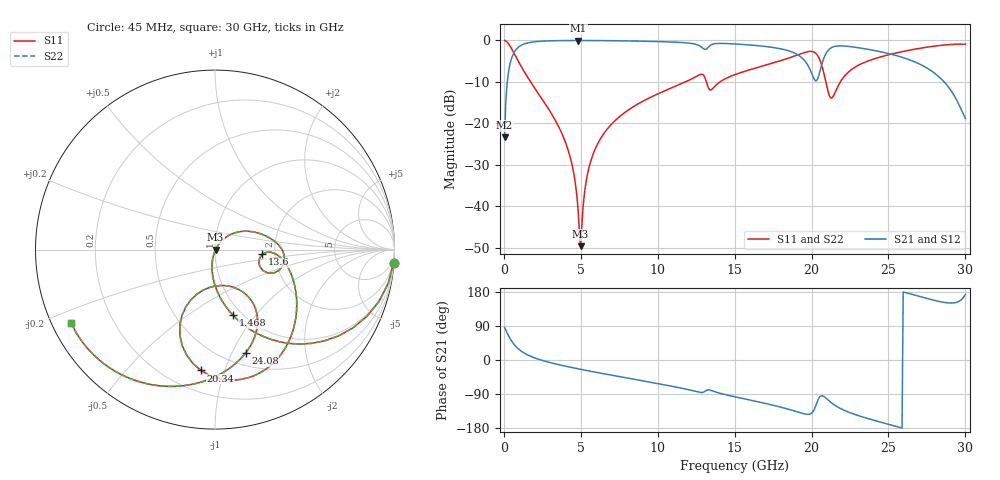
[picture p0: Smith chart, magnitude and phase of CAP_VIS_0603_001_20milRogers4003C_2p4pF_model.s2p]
! S-parameter model data by Modelithics Inc.  support@modelithics.com  813-866-6335  Tampa FL USA
! S-Parameter data specifications:
! Substrate: 20-mil Rogers 4003C, substrate thickness, H=0.508mm, Dielectric constant, Er=3.75
! PCB Mounting Pad Footprint: Pad width, PadW=0.90mm , Pad length, PadL=1.00mm , Pad gap, PadG (edge-to-edge)=1.00mm , Reference planes=3.0mm apart
! Created Wed Nov 18 13:20:45 2015
# hz S ma R 50
! 2 Port Network Data from SP1.SP block
! freq  magS11  angS11  magS21  angS21  magS12  angS12  magS22  angS22
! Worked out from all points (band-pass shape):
!   401 points, 45 MHz to 30 GHz, reference 50 ohm
!   highest |S21| = -0.03 dB at 4.838 GHz (marker M1); lowest = -23.3 dB at 45 MHz (marker M2)
!   |S21| within 3 dB of the highest: 643.6 MHz to 18.88 GHz (18.24 GHz wide, 187 % of centre); 20.96 GHz to 24.84 GHz (3.883 GHz wide, 17 % of centre)
!   lowest |S11| = -49.6 dB at 4.988 GHz (marker M3), VSWR 1.01, Z = 50.3 - j0.0744 ohm
!   |S11| at or under -10 dB: 1.735 GHz to 11.8 GHz (10.07 GHz wide, 149 % of centre); 13.16 GHz to 14.05 GHz (882 MHz wide, 6.48 % of centre); 20.93 GHz to 21.87 GHz (945 MHz wide, 4.42 % of centre)
!   |S22| runs from -49.6 to 0.0 dB; largest |S21 - S12| = 0
!   S11 on the Smith chart (normalised r, x): 45 MHz: 1, -28; 1.468 GHz: 0.91, -0.77; 13.6 GHz: 1.72, -0.10; 20.34 GHz: 0.33, -0.83; 24.08 GHz: 0.63, -1.13; 30 GHz: 0.06, -0.24
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4.5e7  0.9977 -4.1  0.0684 85.9  0.0684 85.9  0.9977 -4.1
4.94325e8  0.7957 -39.7  0.605 50.3  0.605 50.3  0.7957 -39.7
1.467862e9  0.3786 -74.7  0.9238 15.0  0.9238 15.0  0.3786 -74.7
4.014038e9  0.05835 -103.6  0.9951 -16.4  0.9951 -16.4  0.05835 -103.6
4.53825e9  0.02519 -103.8  0.9962 -20.9  0.9962 -20.9  0.02519 -103.8
4.8378e9  0.008286 -90.6  0.9963 -23.3  0.9963 -23.3  0.008286 -90.6
4.987575e9  0.003329 -12.8  0.9963 -24.6  0.9963 -24.6  0.003329 -12.8
5.062462e9  0.005781 30.2  0.9963 -25.2  0.9963 -25.2  0.005781 30.2
5.511788e9  0.02847 54.3  0.9957 -28.7  0.9957 -28.7  0.02847 54.3
6.260662e9  0.06467 52.2  0.9936 -34.5  0.9936 -34.5  0.06467 52.2
1.007992e10  0.2301 25.6  0.9663 -62.9  0.9663 -62.9  0.2301 25.6
1.277588e10  0.3894 -6.7  0.8472 -85.5  0.8472 -85.5  0.3894 -6.7
1.359964e10  0.2659 -5.7  0.9024 -82.1  0.9024 -82.1  0.2659 -5.7
1.50225e10  0.3872 -9.4  0.9052 -97.1  0.9052 -97.1  0.3872 -9.4
1.86171e10  0.6219 -45.4  0.7376 -131.3  0.7376 -131.3  0.6219 -45.4
2.003996e10  0.7353 -81.3  0.3874 -138.9  0.3874 -138.9  0.7353 -81.3
2.033951e10  0.6779 -96.6  0.3293 -113.2  0.3293 -113.2  0.6779 -96.6
2.131305e10  0.2023 -81.1  0.8211 -113.5  0.8211 -113.5  0.2023 -81.1
2.408389e10  0.6005 -73.5  0.7551 -159.4  0.7551 -159.4  0.6005 -73.5
2.505742e10  0.6746 -84.3  0.6902 -170.4  0.6902 -170.4  0.6746 -84.3
2.812781e10  0.8595 -123.2  0.3856 156.1  0.3856 156.1  0.8595 -123.2
3e10  0.8996 -152.9  0.1147 173.1  0.1147 173.1  0.8996 -152.9
